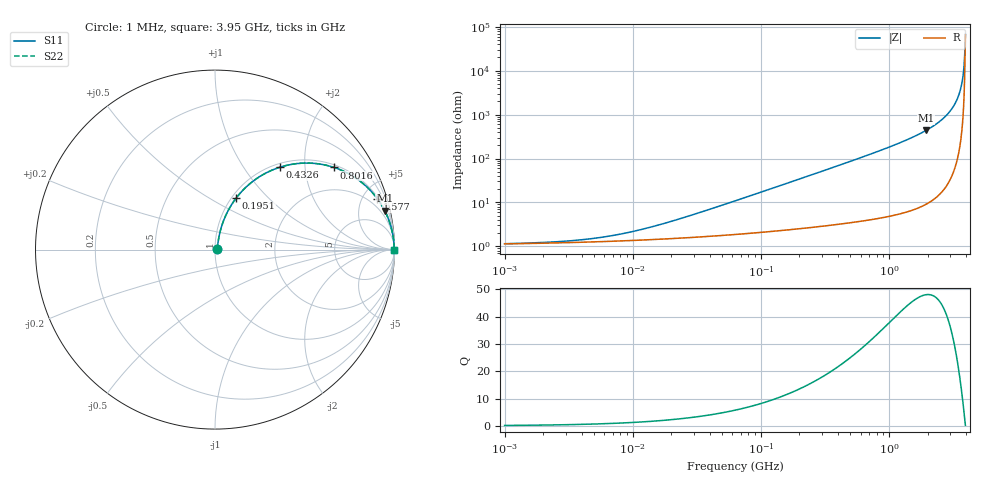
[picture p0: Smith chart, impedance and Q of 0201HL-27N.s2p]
# MHz  S  MA  R  50
!Freq  MagS11  AngS11  MagS21  AngS21  MagS12  AngS12  MagS22  AngS22
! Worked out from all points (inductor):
!   834 points, 1 MHz to 3.95 GHz, reference 50 ohm
!   read as one part in series: L = 27 nH near 28.03 MHz
!   highest Q = 48.1 at 1.943 GHz (marker M1), where L = 35.6 nH
!   S11 on the Smith chart (normalised r, x): 1 MHz: 1.02, +0.00; 195.1 MHz: 1.05, +0.66; 432.6 MHz: 1.07, +1.49; 801.6 MHz: 1.08, +2.84; 1.577 GHz: 1.14, +6.36; 3.95 GHz: open
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1  0.01134 8.4  0.9888 -0.1  0.9888 -0.1  0.01134 8.4
3.987227  0.01394 28.3  0.9877 -0.4  0.9877 -0.4  0.01394 28.3
7.843761  0.01852 44.4  0.9869 -0.8  0.9869 -0.8  0.01852 44.4
15.89798  0.03016 60.3  0.9854 -1.5  0.9854 -1.5  0.03016 60.3
63.38885  0.1066 74.1  0.9763 -6.0  0.9763 -6.0  0.1066 74.1
195.1318  0.3089 67.8  0.9282 -17.9  0.9282 -17.9  0.3089 67.8
250.2433  0.3841 63.8  0.8994 -22.5  0.8994 -22.5  0.3841 63.8
432.5517  0.5845 51.8  0.7862 -35.7  0.7862 -35.7  0.5845 51.8
588.8445  0.7023 43.4  0.687 -44.6  0.687 -44.6  0.7023 43.4
801.6101  0.8061 34.6  0.5682 -53.7  0.5682 -53.7  0.8061 34.6
997.7768  0.8654 28.6  0.4786 -59.9  0.4786 -59.9  0.8654 28.6
1576.945  0.9481 17.3  0.298 -71.4  0.298 -71.4  0.9481 17.3
1943.415  0.9702 12.9  0.2232 -75.9  0.2232 -75.9  0.9702 12.9
2347.857  0.9837 9.2  0.1599 -79.6  0.1599 -79.6  0.9837 9.2
2725.789  0.991 6.5  0.1125 -82.2  0.1125 -82.2  0.991 6.5
3071.487  0.9949 4.3  0.07574 -84.0  0.07574 -84.0  0.9949 4.3
3359.24  0.9969 2.8  0.0487 -85.0  0.0487 -85.0  0.9969 2.8
3565.901  0.9978 1.8  0.03084 -85.1  0.03084 -85.1  0.9978 1.8
3710.691  0.9982 1.1  0.01898 -84.1  0.01898 -84.1  0.9982 1.1
3747.798  0.9983 0.9  0.01603 -83.4  0.01603 -83.4  0.9983 0.9
3938.973  0.9985 0.1  0.001856 -37.7  0.001856 -37.7  0.9985 0.1
3950  0.9985 0.0  0.001493 -11.8  0.001493 -11.8  0.9985 0.0
